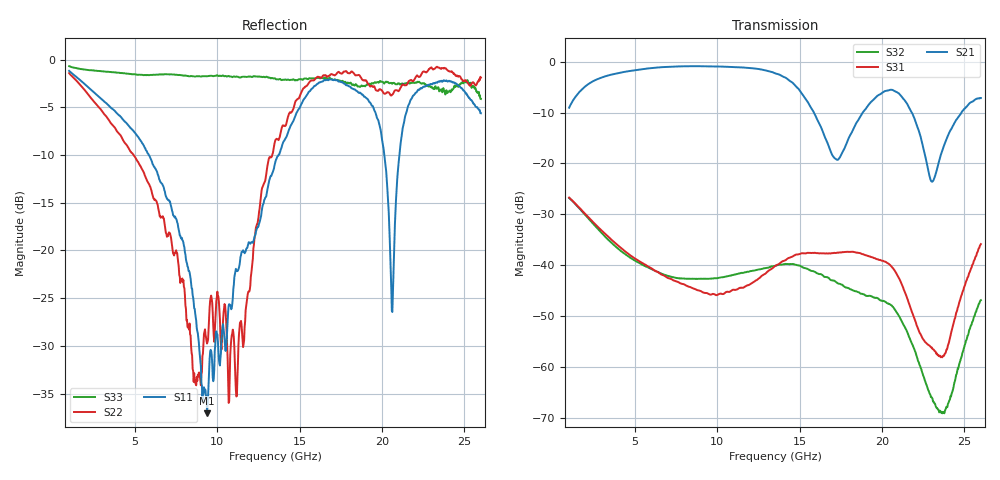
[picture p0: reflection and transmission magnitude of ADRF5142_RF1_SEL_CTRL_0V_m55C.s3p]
! Device: ADRF5142
! Description: Silicon, SPDT Switch, Reflective
! Frequency: 8.00 GHz - 11.00 GHz
! Ports:
!  RFC = Port 1
!  RF1 = Port 2
!  RF2 = Port 3
! VDD = +3.3V
! VSS = -3.3V
! CTRL = 0V
! Temp = -55C
! Data:  Data was collected using an calibrated 4 port network analyzer.
!  The reference plane is the package pins of ADRF5142 switch.
! Notes: Analog Devices supplies this data as a sample of measured data
!  for this product.  Your particular data for this product may vary.
!  Data was taken at -55 degrees C.
!  Analog Devices reserves the right to change this data at anytime.
# HZ S DB R 50
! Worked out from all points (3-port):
!   801 points, 1 GHz to 26 GHz, reference 50 ohm
!   strongest paths, dB at 1 GHz, 7.25 GHz, 13.5 GHz, 19.75 GHz, 26 GHz:
!     S21: -9.1, -1.0, -2.3, -6.7, -7.1
!     S31: -26.7, -42.8, -40.1, -38.8, -35.8
!     S32: -26.8, -42.3, -40.1, -46.5, -46.8
!   lowest |S11| = -37.1 dB at 9.375 GHz (marker M1), VSWR 1.03, Z = 49 + j0.933 ohm
!   |S11| at or under -10 dB: 5.841 GHz to 13.71 GHz (7.869 GHz wide, 80.5 % of centre); 20.14 GHz to 21.05 GHz (913.2 MHz wide, 4.43 % of centre)
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1e9  -1.17 158.8  -9.05 39.3  -26.72 -42.6
     -9.05 39.3  -1.41 123.5  -26.76 -61.3
     -26.72 -42.6  -26.76 -61.3  -0.68 169.2
2.875e9  -3.96 131.1  -3.24 -16.0  -32.85 -88.9
         -3.24 -16.0  -5.12 34.2  -33.31 -143.1
         -32.85 -88.9  -33.31 -143.1  -1.21 153.2
5.875e9  -10.07 96.5  -1.31 -87.4  -40.37 -118.0
         -1.31 -87.4  -13.12 -77.2  -40.55 138.4
         -40.37 -118.0  -40.55 138.4  -1.62 128.2
9.375e9  -37.06 137.2  -0.90 -167.2  -45.46 -131.2
         -0.90 -167.2  -29.75 74.6  -42.62 65.4
         -45.46 -131.2  -42.62 65.4  -1.74 97.8
1.35e10  -10.87 -95.6  -2.27 87.6  -40.14 -147.5
         -2.27 87.6  -8.57 50.5  -40.10 -35.5
         -40.14 -147.5  -40.10 -35.5  -1.96 64.2
1.77812e10  -2.61 153.8  -16.58 73.2  -37.37 117.7
            -16.58 73.2  -1.21 -94.7  -44.31 177.7
            -37.37 117.7  -44.31 177.7  -2.33 22.8
2.05937e10  -26.32 -15.8  -5.52 0.1  -40.33 41.6
            -5.52 0.1  -3.71 -149.0  -47.92 62.9
            -40.33 41.6  -47.92 62.9  -2.51 -6.2
2.20625e10  -3.45 168.7  -12.06 -64.1  -51.33 20.9
            -12.06 -64.1  -1.78 -168.2  -57.43 -14.0
            -51.33 20.9  -57.43 -14.0  -2.38 -24.9
2.36562e10  -2.32 93.6  -17.45 11.9  -58.06 106.7
            -17.45 11.9  -0.88 156.4  -69.06 -88.9
            -58.06 106.7  -69.06 -88.9  -3.42 -46.9
2.6e10  -5.62 7.8  -7.14 -43.2  -35.83 150.9
        -7.14 -43.2  -1.88 96.3  -46.84 126.3
        -35.83 150.9  -46.84 126.3  -4.12 -53.8
